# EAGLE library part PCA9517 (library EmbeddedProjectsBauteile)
I²C Bus Repeater
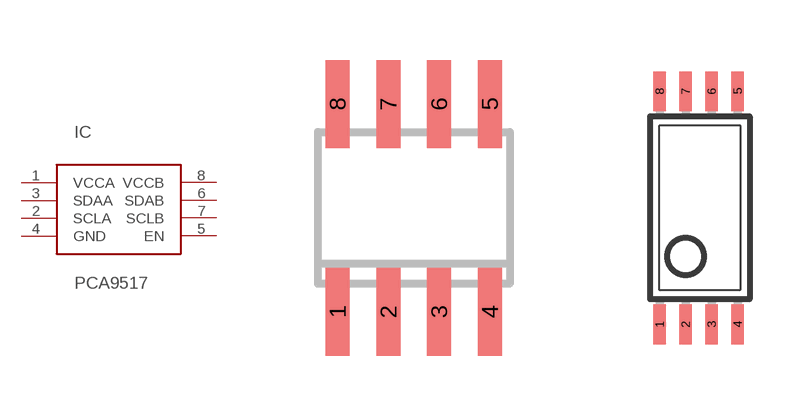
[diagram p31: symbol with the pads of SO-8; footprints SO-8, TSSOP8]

Designator prefix IC

## PCA9517D  [SO-8]
1  VCCA
2  SCLA
3  SDAA
4  GND
5  EN
6  SDAB
7  SCLB
8  VCCB

## PCA9517DP  [TSSOP8]
Pads as for SO-8

## Footprint SO-8 (pad centres in mm)
smd 0.6 x 2.2: 1 -1.905,-2.6; 2 -0.635,-2.6; 3 0.635,-2.6; 4 1.905,-2.6; 5 1.905,2.6; 6 0.635,2.6; 7 -0.635,2.6; 8 -1.905,2.6

## Footprint TSSOP8 (pad centres in mm)
smd 0.305 x 0.991: 1 -1.005,-2.918; 2 -0.355,-2.918; 3 0.295,-2.918; 4 0.945,-2.918; 5 0.945,2.918; 6 0.295,2.918; 7 -0.355,2.918; 8 -1.005,2.918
